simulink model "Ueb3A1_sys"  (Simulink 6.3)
settings: Solver=ode45  StartTime=0.0  StopTime=50  RelTol=1e-3
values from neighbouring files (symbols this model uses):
  T_dach = T    (= 2)    [Ueb3A1.m]
  T_real = 1.0*T    (= 2)    [Ueb3A1.m]
libraries: cstblocks x4

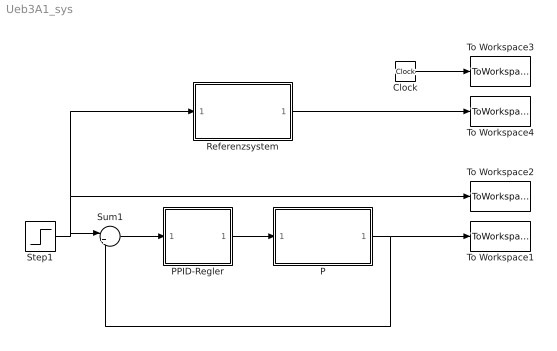
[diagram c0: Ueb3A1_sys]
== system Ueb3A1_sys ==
  Clock : Clock
  P : Subsystem
  PPID-Regler : Subsystem
  Referenzsystem : Subsystem
  Step1 : Step  SampleTime=0
  Sum1 : Sum  Inputs=|+-
  To Workspace1 : ToWorkspace  VariableName=y  SampleTime=-1  SaveFormat=Array
  To Workspace2 : ToWorkspace  VariableName=r  SampleTime=-1  SaveFormat=Array
  To Workspace3 : ToWorkspace  VariableName=t  SampleTime=-1  SaveFormat=Array
  To Workspace4 : ToWorkspace  VariableName=yref  SampleTime=-1  SaveFormat=Array
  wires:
  P/1(y) -> To Workspace1/1, Sum1/2
  Step1/1 -> Sum1/1, Referenzsystem/1(u), To Workspace2/1
  Sum1/1 -> PPID-Regler/1(e)
  PPID-Regler/1(u) -> P/1(u)
  Clock/1 -> To Workspace3/1
  Referenzsystem/1(y) -> To Workspace4/1

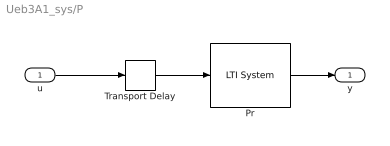
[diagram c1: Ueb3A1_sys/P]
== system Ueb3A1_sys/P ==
  u : Inport
  Pr : cstblocks/LTI System  sys=Pr  IC=[]
  Transport Delay : TransportDelay  DelayTime=T_real
  y : Outport
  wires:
  Transport Delay/1 -> Pr/1
  u/1 -> Transport Delay/1
  Pr/1 -> y/1

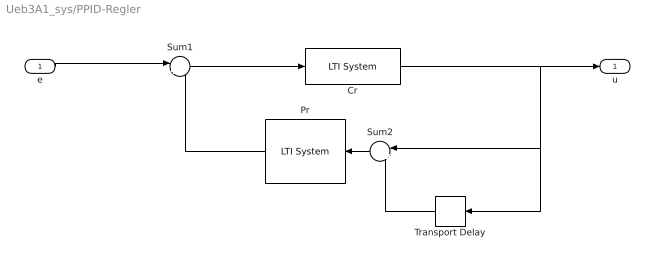
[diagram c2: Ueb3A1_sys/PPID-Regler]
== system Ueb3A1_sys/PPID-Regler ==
  e : Inport
  Cr : cstblocks/LTI System  sys=Cr  IC=[]
  Pr : cstblocks/LTI System  Orientation=left  sys=Pr  IC=[]
  Sum1 : Sum  Inputs=|+-
  Sum2 : Sum  Orientation=left  Inputs=|+-
  Transport Delay : TransportDelay  Orientation=left  DelayTime=T_dach
  u : Outport
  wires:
  Sum1/1 -> Cr/1
  Pr/1 -> Sum1/2
  Transport Delay/1 -> Sum2/2
  Sum2/1 -> Pr/1
  e/1 -> Sum1/1
  Cr/1 -> Sum2/1, Transport Delay/1, u/1

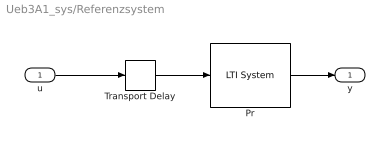
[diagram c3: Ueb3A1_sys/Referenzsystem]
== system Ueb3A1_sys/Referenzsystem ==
  u : Inport
  Pr : cstblocks/LTI System  sys=Tref0  IC=[]
  Transport Delay : TransportDelay  DelayTime=T_real
  y : Outport
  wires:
  Pr/1 -> y/1
  u/1 -> Transport Delay/1
  Transport Delay/1 -> Pr/1
